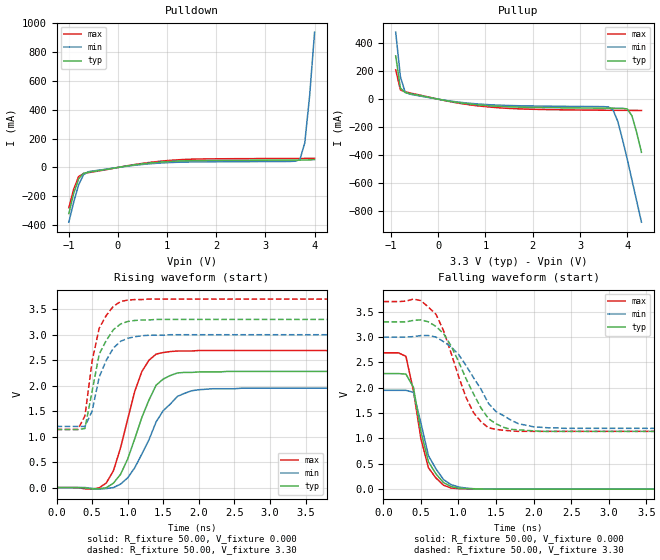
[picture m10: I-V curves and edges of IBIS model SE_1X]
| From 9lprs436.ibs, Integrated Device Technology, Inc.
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|   Model SE_1X
[Model]   SE_1X
Model_type   Output
Polarity   Inverting
Vmeas =   1.50V
Cref =   5.00pF
Rref =  0.000
Vref =   1.50V
C_comp   3.40pF   2.85pF   3.95pF
[Temperature Range]   27.00   70.00   0.000
[Voltage Range]   3.30V   3.00V   3.70V
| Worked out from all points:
|   slope of the pulldown table from 0 to 0.495 V, typ, clamps not added: 20 ohm
|   slope of the pullup table from 0 to 0.495 V, typ, clamps not added: 18 ohm
|   rising waveform, R_fixture 50.00, V_fixture 0.000: 20-80 % time 371ps typ, 438ps min, 321ps max; typ from 0 V to 2.28 V
|   rising waveform, R_fixture 50.00, V_fixture 3.30: 20-80 % time 235ps typ, 249ps min, 201ps max; typ from 1.14 V to 3.3 V
|   falling waveform, R_fixture 50.00, V_fixture 0.000: 20-80 % time 214ps typ, 247ps min, 210ps max; typ from 2.28 V to 0 V
|   falling waveform, R_fixture 50.00, V_fixture 3.30: 20-80 % time 429ps typ, 472ps min, 371ps max; typ from 3.3 V to 1.14 V
[Pulldown]
| voltage   I(typ)   I(min)   I(max)
|  -3.30   -4.16A   -4.01A   -4.26A
|  -3.10   -3.82A   -3.69A   -3.90A
|  -2.90   -3.48A   -3.37A   -3.55A
|  -2.70   -3.14A   -3.04A   -3.20A
|  -2.50   -2.80A   -2.72A   -2.85A
|  -2.30   -2.46A   -2.40A   -2.50A
|  -2.10   -2.12A   -2.09A   -2.15A
|  -1.90   -1.79A   -1.77A   -1.80A
|  -1.70   -1.45A   -1.45A   -1.45A
|  -1.50   -1.12A   -1.14A   -1.10A
-1V       -320mA     -380mA     -280mA
-900mV    -180mA     -240mA     -150mA
-800mV    -79.26mA   -120mA     -62.53mA
-700mV    -40.34mA   -50.05mA   -42.37mA
-600mV    -32.65mA   -29.46mA   -36.03mA
400mV     20.75mA    17.51mA    23.56mA
1.2V      44.23mA    36mA       52.73mA
3.5V      50.96mA    41.9mA     62.28mA
3.7V      51.28mA    53.75mA    62.57mA
3.8V      51.62mA    170mA      62.73mA
3.9V      52.38mA    500mA      62.92mA
4V        54.68mA    940mA      63.14mA
|   4.10   88.45mA   1.41A   63.40mA
|   4.20   0.34A   1.90A   63.77mA
|   4.30   0.77A   2.40A   64.44mA
|   4.50   1.78A   3.42A   76.50mA
|   4.70   2.84A   4.45A   0.67A
|   4.90   3.93A   5.49A   1.70A
|   5.10   5.03A   6.54A   2.81A
|   5.30   6.14A   7.60A   3.94A
|   5.50   7.26A   8.65A   5.08A
|   5.70   8.37A   9.71A   6.23A
|   5.90   9.49A   10.77A   7.38A
|   6.10   10.61A   11.83A   8.54A
|   6.60   13.43A   14.50A   11.45A
[Pullup]
| voltage   I(typ)   I(min)   I(max)
|  -3.30   13.35A   12.84A   13.68A
|  -3.10   12.23A   11.78A   12.52A
|  -2.90   11.10A   10.72A   11.35A
|  -2.70   9.99A   9.66A   10.19A
|  -2.50   8.87A   8.60A   9.04A
|  -2.30   7.75A   7.55A   7.88A
|  -2.10   6.64A   6.50A   6.73A
|  -1.90   5.53A   5.45A   5.58A
|  -1.70   4.43A   4.41A   4.44A
|  -1.50   3.33A   3.38A   3.30A
|  -1.00   0.73A   0.90A   0.61A
-900mV    310mA      480mA      210mA
-800mV    79.51mA    160mA      66.31mA
-700mV    47.89mA    49.75mA    52.51mA
-600mV    40.26mA    36.18mA    44.92mA
300mV     -17.95mA   -15.41mA   -20.73mA
1.1V      -47.43mA   -39.9mA    -56.57mA
3.5V      -64.11mA   -53.44mA   -78.91mA
3.7V      -64.52mA   -77.99mA   -79.38mA
3.8V      -64.75mA   -160mA     -79.6mA
4V        -69.78mA   -430mA     -80.02mA
4.1V      -120mA     -580mA     -80.22mA
4.3V      -380mA     -880mA     -80.81mA
|   4.50   -0.69A   -1.19A   -0.10A
|   4.70   -1.02A   -1.51A   -0.35A
|   4.90   -1.35A   -1.82A   -0.68A
|   5.10   -1.68A   -2.14A   -1.01A
|   5.30   -2.02A   -2.46A   -1.36A
|   5.50   -2.36A   -2.78A   -1.70A
|   5.70   -2.70A   -3.10A   -2.05A
|   5.90   -3.03A   -3.42A   -2.40A
|   6.10   -3.37A   -3.74A   -2.75A
|   6.60   -4.22A   -4.55A   -3.63A
[Ramp]
| variable   typ   min   max
dV/dt_r   1.37/0.36n   1.17/0.45n   1.61/0.31n
dV/dt_f   1.30/0.43n   1.08/0.49n   1.54/0.36n
[Rising Waveform]
R_fixture = 50.00
V_fixture = 0.000
V_fixture_min = 0.000
V_fixture_max = 0.000
| time   V(typ)   V(min)   V(max)
0s        0V         2.37uV     0V
700ps     -2.95mV    -19.38mV   90.43mV
800ps     87.1mV     -120uV     330mV
900ps     260mV      68.14mV    780mV
1.1ns     960mV      390mV      1.89V
1.2ns     1.38V      660mV      2.28V
1.4ns     2.01V      1.29V      2.62V
1.7ns     2.25V      1.79V      2.68V
2ns       2.27V      1.92V      2.69V
5ns       2.28V      1.95V      2.69V
[Rising Waveform]
R_fixture = 50.00
V_fixture = 3.30
V_fixture_min = 3.00
V_fixture_max = 3.70
| time   V(typ)   V(min)   V(max)
0s        1.14V      1.2V       1.14V
300ps     1.14V      1.2V       1.14V
400ps     1.16V      1.2V       1.41V
500ps     1.89V      1.5V       2.48V
600ps     2.62V      2.17V      3.13V
800ps     3.1V       2.74V      3.56V
900ps     3.21V      2.87V      3.65V
1.2ns     3.29V      2.98V      3.69V
1.6ns     3.3V       3V         3.7V
5ns       3.3V       3V         3.7V
[Falling Waveform]
R_fixture = 50.00
V_fixture = 0.000
V_fixture_min = 0.000
V_fixture_max = 0.000
| time   V(typ)   V(min)   V(max)
0s        2.28V      1.95V      2.69V
200ps     2.28V      1.95V      2.69V
300ps     2.27V      1.95V      2.62V
400ps     2.01V      1.91V      1.94V
500ps     1.13V      1.3V       990mV
600ps     540mV      660mV      420mV
800ps     130mV      190mV      78.45mV
900ps     52.74mV    91.15mV    22.63mV
1.4ns     1.98mV     3.33mV     1.17mV
5ns       -3.86uV    2.47uV     2.88uV
[Falling Waveform]
R_fixture = 50.00
V_fixture = 3.30
V_fixture_min = 3.00
V_fixture_max = 3.70
| time   V(typ)   V(min)   V(max)
0s        3.3V       3V         3.7V
500ps     3.34V      3.03V      3.72V
700ps     3.21V      3V         3.45V
900ps     2.83V      2.81V      2.69V
1.1ns     2.18V      2.44V      1.81V
1.2ns     1.88V      2.2V       1.51V
1.4ns     1.39V      1.69V      1.21V
1.7ns     1.18V      1.36V      1.15V
2ns       1.15V      1.23V      1.14V
5ns       1.14V      1.2V       1.14V
